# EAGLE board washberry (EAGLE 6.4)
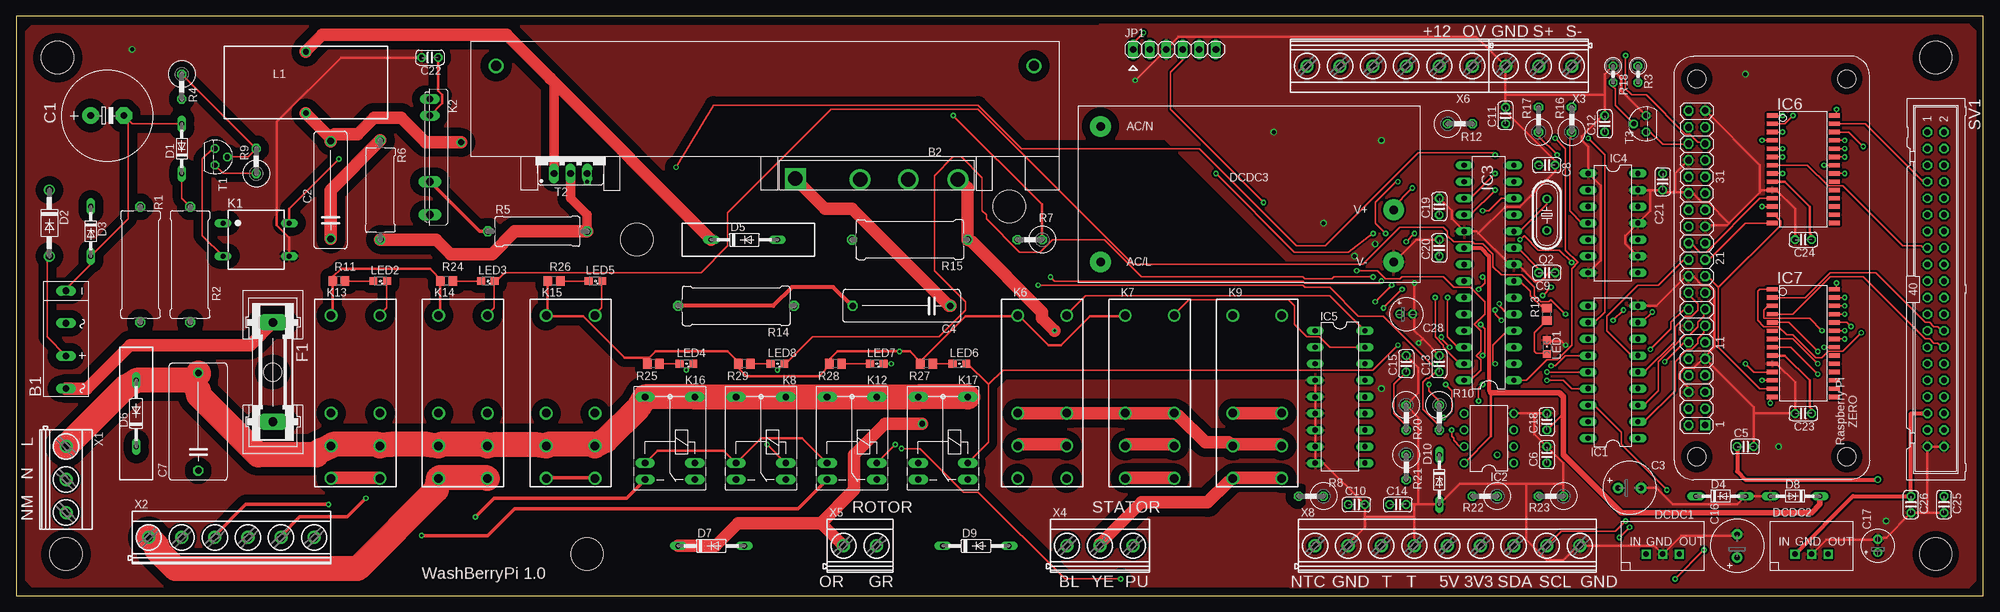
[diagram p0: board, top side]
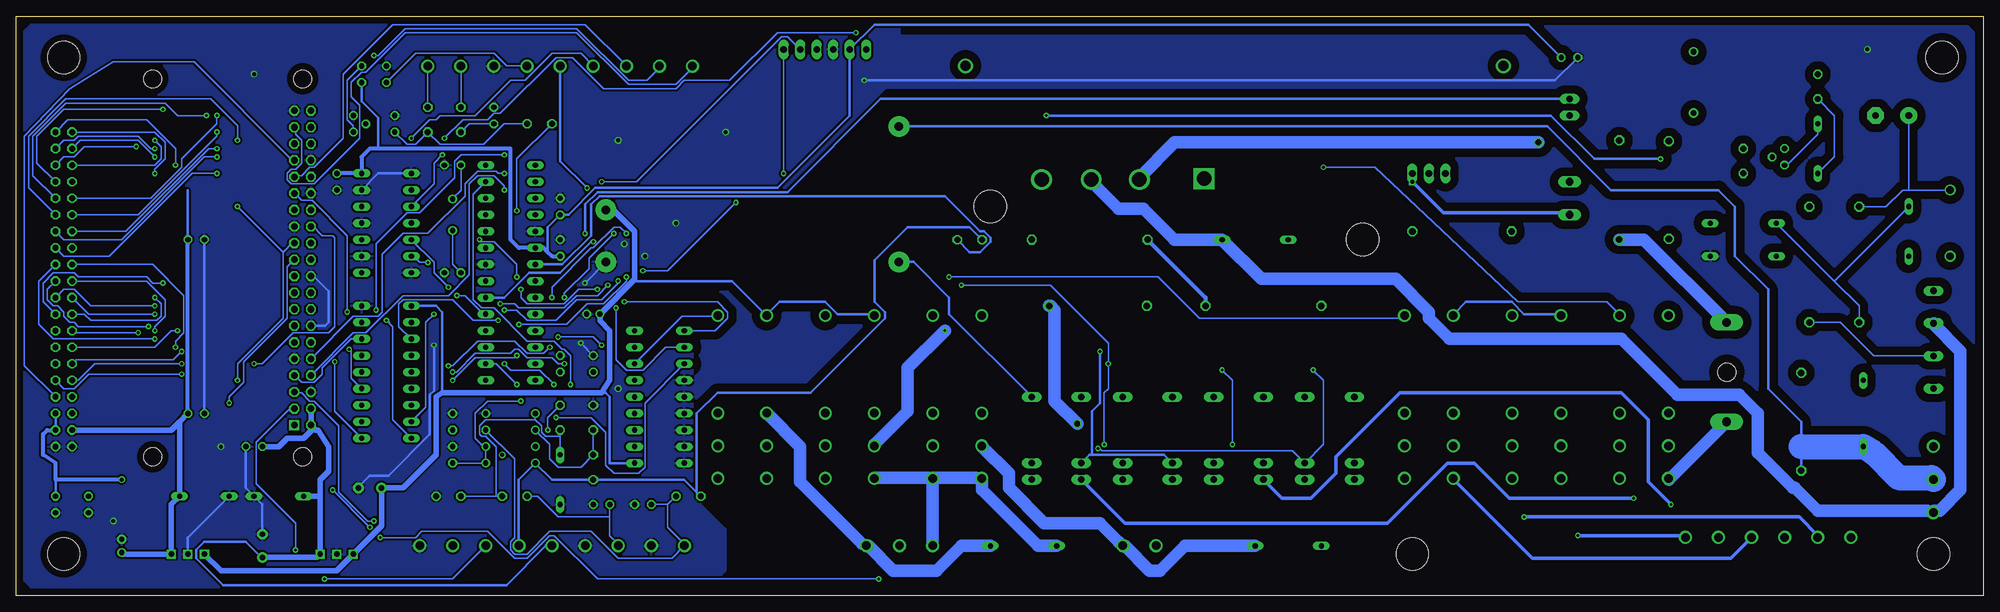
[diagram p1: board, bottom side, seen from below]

Size 301.93 x 88.89 mm. Coordinates in mm from the lower left corner, seen from the top.
Outline: 0,0 301.93,0 301.93,88.89 0,88.89 0,0
Copper layers (1*16): Top 0.035mm / dielectric 1.5mm / Bottom 0.035mm
Design rules "default *": minimum track width 5mil, minimum drill 0.4mm, track to track 6mil, track to pad 6mil, pad to pad 6mil, via to via 6mil, smd to smd 6mil, copper to edge 40mil, drill to drill 8mil, minimum pad ring 10mil, minimum via ring 8mil, stop-mask expansion 4mil, vias tented up to drill 0mil, thermal gap 10mil
Net classes: 0 default: width 0.254 mm; 1 10A: width 3.81 mm, drill 0.001 mm, clearance 1.016 mm; 2 5A: width 1.905 mm, drill 0.001 mm, clearance 1.016 mm; 3 2A: width 0.635 mm, drill 0.001 mm, clearance 1.016 mm; 4 0.5: width 0.508 mm, drill 0.001 mm, clearance 1.016 mm; 5 0.25: width 0.254 mm, clearance 1.016 mm; 6 12V: width 0.406 mm; 7 5V: width 0.406 mm; 8 3V3: width 0.406 mm; 9 small_signal: width 0.203 mm; 10 GND: width 0.406 mm; 11 TRIAC: width 0.406 mm
Holes 5 mm at 6.35,82.55 7.62,6.35 294.64,6.35 294.64,82.55 95.25,54.61 152.4,59.69 87.63,6.35

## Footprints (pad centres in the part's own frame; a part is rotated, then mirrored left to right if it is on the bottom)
2KBB = drill 1.016 long: + -2.616,0; - 7.391,0; AC1 -7.62,0; AC2 2.413,0
5S = drill 2.2 square: + 2.49,1.69 | drill 2.2: - 27.44,1.54; AC1 12.45,1.54; AC2 19.82,1.54
E5-13 = drill 1.016 pad 2.54: + -2.54,0 | drill 1.016 pad 2.54 octagon: - 2.54,0
C150-054X183 = drill 1.016 octagon: 1 -7.493,0; 2 7.493,0
E3,5-8 = drill 0.813 pad 1.6: + -1.778,0 | drill 0.813 pad 1.6 octagon: - 1.778,0
C025-024X044 = drill 0.813 octagon: 1 -1.27,0; 2 1.27,0
C150-091X182 = drill 1.016 octagon: 1 -7.493,0; 2 7.493,0
E2-5 = drill 0.813 pad 1.27: + -1.016,0 | drill 0.813 pad 1.27 octagon: - 1.016,0
DO34Z7 = drill 0.813 long: A 3.81,0; C -3.81,0
DO41-10 = drill 1.118: A 5.08,0; C -5.08,0
DO35-10 = drill 0.813 long: A 5.08,0; C -5.08,0
SIPTO220 = drill 0.813 pad 1.397 square: 1 -2.54,-1.27; 2 0,-1.27; 3 2.54,-1.27
IRM_15/20 = drill 1.3 pad 3.17: AC/L -22.8,-10.4; AC/N -22.8,10.4; V+ 22.2,-2.4; V- 22.2,-10.4
GSH15 = drill 1.321 pad 2.54 long: 1 -7.62,0; 2 7.62,0 | hole 2.794: 0,0
DIL18 = drill 0.813 long: 1 -10.16,-3.81; 2 -7.62,-3.81; 3 -5.08,-3.81; 4 -2.54,-3.81; 5 0,-3.81; 6 2.54,-3.81; 7 5.08,-3.81; 8 7.62,-3.81; 9 10.16,-3.81; 10 10.16,3.81; 11 7.62,3.81; 12 5.08,3.81; 13 2.54,3.81; 14 0,3.81; 15 -2.54,3.81; 16 -5.08,3.81; 17 -7.62,3.81; 18 -10.16,3.81
DIL08 = drill 0.813 pad 1.27: 1 -3.81,-3.81; 2 -1.27,-3.81; 3 1.27,-3.81; 4 3.81,-3.81; 5 3.81,3.81; 6 1.27,3.81; 7 -1.27,3.81; 8 -3.81,3.81
DIL28-3 = drill 0.813 long: 1 -16.51,-3.81; 2 -13.97,-3.81; 3 -11.43,-3.81; 4 -8.89,-3.81; 5 -6.35,-3.81; 6 -3.81,-3.81; 7 -1.27,-3.81; 8 1.27,-3.81; 9 3.81,-3.81; 10 6.35,-3.81; 11 8.89,-3.81; 12 11.43,-3.81; 13 13.97,-3.81; 14 16.51,-3.81; 15 16.51,3.81; 16 13.97,3.81; 17 11.43,3.81; 18 8.89,3.81; 19 6.35,3.81; 20 3.81,3.81; 21 1.27,3.81; 22 -1.27,3.81; 23 -3.81,3.81; 24 -6.35,3.81; 25 -8.89,3.81; 26 -11.43,3.81; 27 -13.97,3.81; 28 -16.51,3.81
DIL14 = drill 0.813 long: 1 -7.62,-3.81; 2 -5.08,-3.81; 3 -2.54,-3.81; 4 0,-3.81; 5 2.54,-3.81; 6 5.08,-3.81; 7 7.62,-3.81; 8 7.62,3.81; 9 5.08,3.81; 10 2.54,3.81; 11 0,3.81; 12 -2.54,3.81; 13 -5.08,3.81; 14 -7.62,3.81
SO28W = smd 0.65 x 1.7: 1 -7.62,-4.78; 2 -6.35,-4.78; 3 -5.08,-4.78; 4 -3.81,-4.78; 5 -2.54,-4.78; 6 -1.27,-4.78; 7 0,-4.78; 8 1.27,-4.78; 9 2.54,-4.78; 10 3.81,-4.78; 11 5.08,-4.78; 12 6.35,-4.78; 13 7.62,-4.78; 14 8.89,-4.78; 15 8.89,4.78; 16 7.62,4.78; 17 6.35,4.78; 18 5.08,4.78; 19 3.81,4.78; 20 2.54,4.78; 21 1.27,4.78; 22 0,4.78; 23 -1.27,4.78; 24 -2.54,4.78; 25 -3.81,4.78; 26 -5.08,4.78; 27 -6.35,4.78; 28 -7.62,4.78
1X06 = drill 1.016 long: 1 -6.35,0; 2 -3.81,0; 3 -1.27,0; 4 1.27,0; 5 3.81,0; 6 6.35,0
AQY27 = drill 0.8 long: 1 -2.54,-5.08; 2 2.54,-5.08; 3 2.54,5.08; 4 -2.54,5.08
AQZ-SIL04 = drill 1 long: 1 -8.89,0; 2 -6.35,0 | drill 1.2 long: 3 3.81,0; 4 8.89,0
FTR-K1C = drill 1.3 pad 1.93: 1 -12.5,-3.75; 2 2.5,-3.75; 3 7.5,-3.75; 4 12.5,-3.75; 5 12.5,3.75; 6 7.5,3.75; 7 2.5,3.75; 8 -12.5,3.75
M3XXH = drill 1.016 long: 1 -3.81,3.81; 2 -3.81,-3.81; O -6.35,-3.81; P 6.35,-3.81; P@ 6.35,3.81; S -6.35,3.81
TJ5-U1 = drill 0.9: 1 -4.7,0; 2 4.7,0
CHIPLED_0805 = smd 1.2 x 1.2: A 0,-1.05; C 0,1.05
SML0805 = smd 1.2 x 1.2: A 1.05,0; C -1.05,0
HC49/S = drill 0.813: 1 -2.413,0; 2 2.413,0
0617/17 = drill 1.016 octagon: 1 -8.89,0; 2 8.89,0
0207/2V = drill 0.813 octagon: 1 -1.27,0; 2 1.27,0
0411V = drill 0.914 octagon: 1 -2.54,0; 2 1.27,0
P0613/15 = drill 1.016 octagon: 1 -7.62,0; 2 7.62,0
R0805 = smd 1.3 x 1.5: 1 -0.95,0; 2 0.95,0
W_HEATSINK = drill 1.5: P$1 -40.64,5.08; P$2 41.91,5.08
ML40 = drill 0.914 octagon: 1 -24.13,-1.27; 2 -24.13,1.27; 3 -21.59,-1.27; 4 -21.59,1.27; 5 -19.05,-1.27; 6 -19.05,1.27; 7 -16.51,-1.27; 8 -16.51,1.27; 9 -13.97,-1.27; 10 -13.97,1.27; 11 -11.43,-1.27; 12 -11.43,1.27; 13 -8.89,-1.27; 14 -8.89,1.27; 15 -6.35,-1.27; 16 -6.35,1.27; 17 -3.81,-1.27; 18 -3.81,1.27; 19 -1.27,-1.27; 20 -1.27,1.27; 21 1.27,-1.27; 22 1.27,1.27; 23 3.81,-1.27; 24 3.81,1.27; 25 6.35,-1.27; 26 6.35,1.27; 27 8.89,-1.27; 28 8.89,1.27; 29 11.43,-1.27; 30 11.43,1.27; 31 13.97,-1.27; 32 13.97,1.27; 33 16.51,-1.27; 34 16.51,1.27; 35 19.05,-1.27; 36 19.05,1.27; 37 21.59,-1.27; 38 21.59,1.27; 39 24.13,-1.27; 40 24.13,1.27
TO92 = drill 0.813 octagon: 1 1.27,0; 2 0,1.905; 3 -1.27,0
TO220BV = drill 1.016 long: G 2.54,-2.54; T1 -2.54,-2.54; T2 0,-2.54
ZERO_NO_DIMENSION = drill 1.016 square: 1 8.37,25.24 | drill 1.016 octagon: 2 8.37,27.78; 3 10.91,25.24; 4 10.91,27.78; 5 13.45,25.24; 6 13.45,27.78; 7 15.99,25.24; 8 15.99,27.78; 9 18.53,25.24; 10 18.53,27.78; 11 21.07,25.24; 12 21.07,27.78; 13 23.61,25.24; 14 23.61,27.78; 15 26.15,25.24; 16 26.15,27.78; 17 28.69,25.24; 18 28.69,27.78; 19 31.23,25.24; 20 31.23,27.78; 21 33.77,25.24; 22 33.77,27.78; 23 36.31,25.24; 24 36.31,27.78; 25 38.85,25.24; 26 38.85,27.78; 27 41.39,25.24; 28 41.39,27.78; 29 43.93,25.24; 30 43.93,27.78; 31 46.47,25.24; 32 46.47,27.78; 33 49.01,25.24; 34 49.01,27.78; 35 51.55,25.24; 36 51.55,27.78; 37 54.09,25.24; 38 54.09,27.78; 39 56.63,25.24; 40 56.63,27.78 | hole 2.75: 3.5,3.5; 3.5,26.5; 61.5,26.5; 61.5,3.5
MKDSN1,5/3-5,08 = drill 1.3 pad 2: 1 -7.641,0.025; 2 -2.561,0.025; 3 2.519,0.025
MKDSN1,5/6-5,08 = drill 1.3 pad 2: 1 -12.7,0.025; 2 -7.62,0.025; 3 -2.54,0.025; 4 2.54,0.025; 5 7.62,0.025; 6 12.7,0.025
MKDSN1,5/2-5,08 = drill 1.3 pad 2: 1 -2.561,0.025; 2 2.519,0.025
MKDSN1,5/9-5,08 = drill 1.3 pad 2: 1 -20.341,0.025; 2 -15.261,0.025; 3 -10.181,0.025; 4 -5.101,0.025; 5 -0.021,0.025; 6 5.059,0.025; 7 10.139,0.025; 8 15.219,0.025; 9 20.299,0.025

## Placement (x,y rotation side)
B1  [2KBB]  7.62,39.37 90 top
B2  D15XB60  [5S]  117.1,62.3 0 top
C1  470µ  [E5-13]  13.97,73.66 0 top
C2  1nF  [C150-054X183]  48.26,62.23 90 top
C3  100µF  [E3,5-8]  247.65,16.51 0 top
C4  100nF  [C150-054X183]  135.89,44.45 180 top
C5  100nF  [C025-024X044]  265.43,22.86 0 top
C6  100nF  [C025-024X044]  234.95,21.59 90 top
C7  1nF  [C150-091X182]  27.94,26.67 90 top
C8  20pF  [C025-024X044]  234.95,66.04 0 top
C9  20pF  [C025-024X044]  234.95,49.53 0 top
C10  22nF  [C025-024X044]  205.74,13.97 0 top
C11  100nF  [C025-024X044]  228.6,73.66 90 top
C12  0  [C025-024X044]  243.84,72.39 90 top
C13  22pF  [C025-024X044]  218.44,35.56 90 top
C14  100nF  [C025-024X044]  212.09,13.97 0 top
C15  100nF  [C025-024X044]  213.36,35.56 90 top
C16  100µF  [E3,5-8]  264.16,7.62 90 top
C17  100µF  [E2-5]  285.75,7.62 90 top
C18  100nF  [C025-024X044]  234.95,26.67 90 top
C19  100nF  [C025-024X044]  218.44,59.69 90 top
C20  100nF  [C025-024X044]  218.44,53.34 90 top
C21  100nF  [C025-024X044]  252.73,63.5 270 top
C22  100nF  [C025-024X044]  63.5,82.55 180 top
C23  100nF  [C025-024X044]  274.32,27.94 180 top
C24  100nF  [C025-024X044]  274.32,54.61 180 top
C25  100nF  [C025-024X044]  295.91,13.97 270 top
C26  100nF  [C025-024X044]  290.83,13.97 270 top
C28  [E2-5]  213.36,43.18 0 top
D1  12V  [DO34Z7]  25.4,68.58 90 top
D2  1N4004  [DO41-10]  5.08,57.15 270 top
D3  5V  [DO34Z7]  11.43,55.88 270 top
D4  5V8  [DO34Z7]  261.62,15.24 0 top
D5  [DO35-10]  111.76,54.61 0 top
D6  [DO35-10]  18.41,27.94 90 top
D7  [DO35-10]  106.68,7.62 0 top
D8  3V6  [DO34Z7]  273.05,15.24 180 top
D9  [DO35-10]  147.32,7.62 0 top
D10  3V3  [DO34Z7]  218.44,17.78 270 top
DCDC1  TSR1-2405  [SIPTO220]  252.73,7.62 0 top
DCDC2  TSR1-2405  [SIPTO220]  275.59,7.62 0 top
DCDC3  IRM-15-12  [IRM_15/20]  189.23,61.59 0 top
F1  5A  [GSH15]  39.37,34.29 270 top
IC1  ULN2803  [DIL18]  245.11,34.29 90 top
IC2  LM358N  [DIL08]  226.06,24.13 90 top
IC3  PIC18F2550_28DIP  [DIL28-3]  226.06,49.53 90 top
IC4  74HC04N  [DIL14]  245.11,57.15 270 top
IC5  ULN2803  [DIL18]  203.2,30.48 270 top
IC6  MCP23S17SO  [SO28W]  274.32,66.04 270 top
IC7  MCP23S17SO  [SO28W]  274.32,39.37 270 top
JP1  ISCP  [1X06]  177.8,83.82 0 top
K1  AQYAQY27  [AQY27]  36.83,54.61 270 top
K2  AQZ204  [AQZ-SIL04]  63.5,67.31 270 top
K6  FTR-K1C  [FTR-K1C]  157.48,30.48 270 top
K7  FTR-K1C  [FTR-K1C]  173.99,30.48 270 top
K8  M3XXH  [M3XXH]  114.3,24.13 90 top
K9  FTR-K1C  [FTR-K1C]  190.5,30.48 270 top
K12  M3XXH  [M3XXH]  128.27,24.13 90 top
K13  FTR-K1C  [FTR-K1C]  52.07,30.48 270 top
K14  FTR-K1C  [FTR-K1C]  68.58,30.48 270 top
K15  FTR-K1C  [FTR-K1C]  85.09,30.48 270 top
K16  M3XXH  [M3XXH]  100.33,24.13 90 top
K17  M3XXH  [M3XXH]  142.24,24.13 90 top
L1  [TJ5-U1]  44.45,78.74 270 top
LED1  [CHIPLED_0805]  234.95,38.1 0 top
LED2  [SML0805]  55.88,48.26 180 top
LED3  [SML0805]  72.39,48.26 180 top
LED4  [SML0805]  102.87,35.56 180 top
LED5  [SML0805]  88.9,48.26 180 top
LED6  [SML0805]  144.78,35.56 180 top
LED7  [SML0805]  132.08,35.56 180 top
LED8  [SML0805]  116.84,35.56 180 top
Q2  12MHz  [HC49/S]  234.95,58.42 270 top
R1  82K  [0617/17]  19.05,50.8 270 top
R2  47K  [0617/17]  26.67,50.8 270 top
R3  10K  [0207/2V]  248.92,80.01 270 top
R4  1K  [0411V]  25.4,77.47 270 top
R5  470  [P0613/15]  80.01,55.88 0 top
R6  68  [P0613/15]  55.88,62.23 270 top
R7  1K  [0411V]  154.94,54.61 180 top
R8  10K  [0411V]  198.12,15.24 180 top
R9  47K  [0411V]  36.83,67.31 90 top
R10  10K  [0411V]  218.44,26.67 270 top
R11  [R0805]  49.53,48.26 180 top
R12  1K  [0411V]  222.25,72.39 0 top
R13  1K  [R0805]  234.95,43.18 90 top
R14  68  [0617/17]  110.49,44.45 180 top
R15  68  [0617/17]  137.16,54.61 180 top
R16  0  [0411V]  238.76,73.66 90 top
R17  0  [0411V]  233.68,73.66 90 top
R18  470K  [0207/2V]  245.11,80.01 270 top
R20  1K  [0411V]  213.36,26.67 270 top
R21  8K2  [0411V]  213.36,19.05 270 top
R22  1K  [0411V]  224.79,15.24 180 top
R23  47K  [0411V]  234.95,15.24 180 top
R24  [R0805]  66.04,48.26 180 top
R25  [R0805]  97.79,35.56 180 top
R26  [R0805]  82.55,48.26 180 top
R27  [R0805]  139.7,35.56 180 top
R28  [R0805]  125.73,35.56 180 top
R29  [R0805]  111.76,35.56 180 top
SINK1  HEATSINK  [W_HEATSINK]  114.3,76.2 0 top
SV1  [ML40]  294.64,46.99 270 top
T1  BC547  [TO92]  30.48,67.31 270 top
T2  BTA25-6CWG  [TO220BV]  85.09,67.31 0 top
T3  BC547  [TO92]  250.19,72.39 90 top
U$3  ZERO  [ZERO_NO_DIMENSION]  284.48,17.78 90 top
X1  [MKDSN1,5/3-5,08]  7.62,15.24 270 top
X2  MKDSN1,5/6-5,08  [MKDSN1,5/6-5,08]  33.02,8.89 0 top
X3  MKDSN1,5/3-5,08  [MKDSN1,5/3-5,08]  231.14,81.28 180 top
X4  MKDSN1,5/3-5,08  [MKDSN1,5/3-5,08]  168.91,7.62 0 top
X5  MKDSN1,5/2-5,08  [MKDSN1,5/2-5,08]  129.54,7.62 0 top
X6  MKDSN1,5/6-5,08  [MKDSN1,5/6-5,08]  210.82,81.28 180 top
X8  MKDSN1,5/9-5,08  [MKDSN1,5/9-5,08]  219.71,7.62 0 top

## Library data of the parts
B1 = rectifier
B2 = D15XB60
C1-C26 C28 L1 R1-R18 R20-R29 = rcl
D1-D10 = diode
DCDC1 DCDC2 = TSR1-24XX
DCDC3 = meanwell_irm_v7
F1 = fuse; MPN: 64900001039; OC_FARNELL: 1271673; OC_NEWARK: 02P0318
IC1 IC5 = uln-udn
IC2 = linear
IC3 = microchip; MF: MICROCHIP; MPN: PIC18F2550-I/SP; OC_FARNELL: 1523822; OC_NEWARK: 80K6054
IC4 = 74xx-eu
IC6 IC7 = microchip; MF: MICROCHIP; MPN: MCP23S17-E/SO; OC_FARNELL: unknown; OC_NEWARK: 31K2950
JP1 = pinhead
K1 K6-K9 K12-K17 = relay; OC_FARNELL: unknown; OC_NEWARK: unknown
K2 = relay; MPN: AQZ204; OC_FARNELL: unknown; OC_NEWARK: 13P1222
LED1-LED8 = led
Q2 = crystal; OC_FARNELL: 1667008; OC_NEWARK: unknown
SINK1 = Heatsink_Washmachine
SV1 = con-harting-ml; OC_FARNELL: unknown; OC_NEWARK: unknown
T1 T3 = transistor
T2 = triac
U$3 = RasPiZero
X1 X3 X4 = con-phoenix-508; MPN: SMKDSN1,5/3-5,08; OC_FARNELL: 1792904; OC_NEWARK: 70R0299
X2 X6 = con-phoenix-508; MPN: SMKDSN1,5/6-5,08; OC_FARNELL: 1792907; OC_NEWARK: 70R0302
X5 = con-phoenix-508; MPN: MKDSN 1,5/2-5.08; OC_FARNELL: 1792903; OC_NEWARK: 30M2397
X8 = con-phoenix-508; MPN: SMKDSN1,5/9-5,08; OC_FARNELL: 1792912; OC_NEWARK: 70R0305

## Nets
+3V3 [3V3]: C17.+ C18.1 C19.1 C20.1 C21.1 C22.1 C23.1 C24.1 D8.C DCDC2.3 IC2.8 IC3.20 IC4.14 IC6.9 IC7.9 JP1.2 K2.2 R3.2 R7.2 R8.2 R21.2 SV1.37 X8.6
+5V [5V]: C5.1 C16.+ C25.1 D4.C DCDC1.3 SV1.36 SV1.38 U$3.2 U$3.4 X8.5
+12V [12V]: C3.+ C26.1 C28.+ DCDC1.1 DCDC2.1 DCDC3.V+ IC1.10 IC5.10 K6.1 K7.1 K8.1 K9.1 K12.1 K13.1 K14.1 K15.1 K16.1 K17.1 R11.2 R24.2 R25.2 R26.2 R27.2 R28.2 R29.2 SV1.35 X6.2
BOOST [small_signal]: IC3.4 IC5.3
CS0: IC6.11 U$3.24
CS1: IC7.11 U$3.26
DIRECTION [small_signal]: IC3.5 IC4.5 IC5.1
GND [GND]: C3.- C5.2 C6.2 C8.2 C9.2 C10.2 C11.2 C12.2 C13.2 C14.2 C15.2 C16.- C17.- C18.2 C19.2 C20.2 C21.2 C22.2 C23.2 C24.2 C25.2 C26.2 C28.- D4.A D8.A D10.A DCDC1.2 DCDC2.2 DCDC3.V- IC1.9 IC2.4 IC3.8 IC3.19 IC4.1 IC4.7 IC4.9 IC4.11 IC4.13 IC5.4 IC5.5 IC5.6 IC5.7 IC5.8 IC5.9 IC6.10 IC7.10 JP1.3 K1.3 LED1.C R18.1 R20.1 R23.1 SV1.39 SV1.40 T3.1 U$3.6 U$3.9 U$3.14 U$3.20 U$3.25 U$3.30 U$3.34 U$3.39 X3.3 X8.2 X8.4 X8.9
GPA1.0: IC6.21 SV1.1
GPA1.1: IC6.22 SV1.2
GPA1.2: IC6.23 SV1.3
GPA1.3: IC6.24 SV1.4
GPA1.4: IC6.25 SV1.5
GPA1.5: IC6.26 SV1.6
GPA1.6: IC6.27 SV1.7
GPA1.7: IC6.28 SV1.8
GPA2.0: IC7.21 SV1.17
GPA2.1: IC7.22 SV1.18
GPA2.2: IC7.23 SV1.19
GPA2.3: IC7.24 SV1.20
GPA2.4: IC7.25 SV1.21
GPA2.5: IC7.26 SV1.22
GPA2.6: IC7.27 SV1.23
GPA2.7: IC7.28 SV1.24
GPB1.0: IC6.1 SV1.9
GPB1.1: IC6.2 SV1.10
GPB1.2: IC6.3 SV1.11
GPB1.3: IC6.4 SV1.12
GPB1.4: IC6.5 SV1.13
GPB1.5: IC6.6 SV1.14
GPB1.6: IC6.7 SV1.15
GPB1.7: IC6.8 SV1.16
GPB2.0: IC7.1 SV1.25
GPB2.1: IC7.2 SV1.26
GPB2.2: IC7.3 SV1.27
GPB2.3: IC7.4 SV1.28
GPB2.4: IC7.5 SV1.29
GPB2.5: SV1.30
GPB2.6: IC7.7 SV1.31
GPB2.7: IC7.8 SV1.32
GPIO0: U$3.11
GPIO1 [small_signal]: IC1.1 U$3.12
GPIO2 [small_signal]: IC1.2 U$3.13
GPIO3 [small_signal]: IC1.3 U$3.15
GPIO4 [small_signal]: IC1.4 U$3.16
GPIO5 [small_signal]: IC1.5 U$3.18
GPIO6 [small_signal]: IC1.6 U$3.22
GPIO7 [small_signal]: IC1.7 U$3.7
GPIO21 [small_signal]: IC1.8 U$3.29
GPIO27 [small_signal]: R3.1 T3.3 U$3.36
GPPB2.5: IC7.6
INT [TRIAC]: IC3.21 K1.4 R7.1
L [10A]: C7.2 D6.A DCDC3.AC/L K8.P K8.P@ K12.P K12.P@ K13.3 K13.6 K14.3 K14.6 K15.3 K15.6 K16.P K16.P@ K17.P K17.P@ X1.1
L-MOTOR [5A]: F1.2 K13.4 K13.5
MISO: IC6.14 IC7.14 U$3.21
MOSI: IC6.13 IC7.13 U$3.19
N [10A]: C7.1 D6.C DCDC3.AC/N X1.2
N$1 [0.25]: K1.2 T1.3
N$2 [0.25]: B1.- C1.- D1.A D3.A R9.1 T1.1
N$3 [0.25]: C1.+ D2.C R1.1
N$4 [0.25]: D3.C K1.1 R1.2
N$5 [small_signal]: IC3.7 R13.2
N$6 [small_signal]: LED1.A R13.1
N$7 [0.25]: D1.C R2.1 R4.2
N$8: IC1.11 X6.3
N$9 [0.25]: R4.1 R9.2 T1.2
N$10 [0.25]: B1.+ D2.A R2.2
N$11 [small_signal]: R18.2 T3.2 X6.1
N$12 [0.5]: K2.4 T2.G
N$13 [0.5]: K2.3 R5.1
N$14: IC2.7 IC3.13 R10.1
N$15: IC1.18 K13.8 LED2.C
N$16 [5A]: B2.- K7.3 K7.6 R15.1
N$17 [5A]: C2.1 R6.1
N$18 [5A]: B2.AC1 C2.2 L1.2
N$19: C6.1 IC2.1 IC2.2 IC3.2
N$20 [5A]: K9.4 K9.5 X4.2
N$21 [5A]: D9.A K9.2 K9.7 X4.3
N$22: LED2.A R11.1
N$23 [5A]: D5.C L1.1 T2.T1
N$24 [5A]: B2.+ C4.1 D7.C X5.1
N$25 [small_signal]: C9.1 IC3.9 Q2.2
N$26 [small_signal]: C8.1 IC3.10 Q2.1
N$27 [small_signal]: IC3.12 R12.1
N$28: C11.1 IC4.3 R17.1
N$29: C12.1 IC4.4 R12.2 R16.1
N$30: IC1.17 K14.8 LED3.C
N$31 [2A]: R14.1 R15.2
N$32 [2A]: C4.2 R14.2
N$33 [5A]: K6.2 K6.7 K7.2 K7.7 K9.3 K9.6
N$34 [5A]: D9.C K6.4 K6.5 K7.4 K7.5 X4.1
N$35 [5A]: D7.A K6.3 K6.6 X5.2
N$36: IC5.18 K6.8
N$37: R16.2 X3.1
N$38: R17.2 X3.2
N$39: C15.1 IC2.6 R20.2 R21.1
N$40: LED3.A R24.1
N$41: C13.1 D10.C IC2.5 R10.2 R22.1 R23.2
N$42: IC1.16 K16.2 LED4.C
N$43: U$3.31 X6.4
N$44: U$3.35 X6.5
N$45: LED4.A R25.1
N$46: LED5.A R26.1
N$49: IC1.13 K17.2 LED6.C
N$50: LED6.A R27.1
N$51: IC1.14 K12.2 LED7.C
N$52: LED7.A R28.1
N$53: IC1.15 K8.2 LED8.C
N$54: LED8.A R29.1
N$55: IC1.12 K15.8 LED5.C
N$56: SV1.33
N$57 [small_signal]: IC4.6 IC5.2
N$58: U$3.37 X6.6
N$60: IC5.17 K7.8
N$62: IC5.16 K9.8
N$63 [10A]: K14.4 K14.5 X2.1
N$64 [0.5]: K16.S X2.2
N$65 [0.5]: K8.S X2.3
N$66 [0.5]: K12.S X2.6
N$67 [0.5]: K17.S X2.5
N$68 [0.5]: K15.4 K15.5 X2.4
N_MOTOR [5A]: B1.AC2 B2.AC2 D5.A X1.3
NTC: C10.1 IC2.3 R8.1 X8.1
PGC [small_signal]: IC3.27 JP1.5
PGD [small_signal]: IC3.28 JP1.4
PGM [small_signal]: IC3.26 JP1.6
PWM0: U$3.32
PWM1: SV1.34 U$3.33
RX: IC3.18 U$3.8
SCK: IC6.12 IC7.12 U$3.23
SCL: U$3.5 X8.8
SDA: U$3.3 X8.7
SUPPLY_MOTOR [5A]: B1.AC1 F1.1 R5.2 R6.2 T2.T2
TACHO: C14.1 R22.2 X8.3
TRIAC [TRIAC]: IC3.6 K2.1
TX: IC3.17 U$3.10
VPP [small_signal]: IC3.1 JP1.1

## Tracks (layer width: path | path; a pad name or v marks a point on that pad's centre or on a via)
+3V3
  Top 0.406: 226.38,31.11 226.38,24.45 IC2.8 | C22.1 64.77,77.47 65.41,76.83 65.41,75.56 K2.2 | IC7.9 271.46,36.83 275.27,33.02 275.27,28.89 275.59,28.57 C23.1 | IC6.9 271.46,63.5 275.27,59.69 275.27,55.56 275.59,55.24 C24.1 | C18.1 237.17,27.62 237.49,27.62
  Top 0.61: IC3.20 224.79,53.34 226.06,52.07 226.06,31.43 226.38,31.11
  Top 0.813: 226.38,31.11 236.85,31.11 237.49,30.48 237.49,27.62 237.49,21.59 246.38,12.7 275.59,12.7 276.86,13.97 D8.C
  Bottom 0.406: C24.1 275.59,62.23 | 197.49,15.88 199.39,17.78 R21.2 219.71,17.78 IC2.8 224.79,17.78 224.79,7.94 X8.6 | 197.49,15.88 R8.2 | R7.2 155.57,56.52 165.1,56.52 170.18,51.44 170.18,45.09 168.59,43.5 168.59,42.55 180.02,31.11 194.31,31.11 197.49,27.94 197.49,15.88 | 220.5,52.86 220.34,53.02 220.34,56.52 C19.1 217.17,58.42 213.04,62.55 185.1,62.55 173.99,73.66 JP1.2 170.18,87.63 69.85,87.63 C22.1 | R3.2 248.92,75.88 246.38,73.34 246.38,68.58
  Bottom 0.61: C23.1 C24.1 | C20.1 219.71,52.07 220.5,52.86 220.98,53.34 IC3.20 224.79,53.34 226.06,54.61 226.06,68.58 246.38,68.58 247.65,68.58 248.92,67.31 IC4.14 C21.1
  Bottom 0.813: C17.+ 285.5,6.35 DCDC2.3 278.13,13.97 D8.C 276.86,26.67 | SV1.37 278.13,25.4 276.86,26.67 | 276.86,26.67 C23.1
+5V  (via drill 0.6)
  Top 0.61: C5.1 264.16,19.05 265.43,17.78 v285.75,17.78
  Bottom 0.406: 295.91,17.78 C25.1 | SV1.38 SV1.36 | X8.5 219.71,7.62 220.66,7.62 226.69,1.59 270.19,1.59 274.32,5.71 274.32,6.99 273.05,8.26 266.7,8.26 264.48,6.03 C16.+
  Bottom 0.61: v285.75,17.78 295.91,17.78 295.91,20.32 297.81,21.59 297.81,24.77 297.18,25.4 SV1.38
  Bottom 0.813: 255.27,15.24 DCDC1.3 255.78,5.84 C16.+ | D4.C 255.27,15.24 | 255.27,15.24 255.27,17.78 254,19.05 254,22.86 255.59,25.4 255.95,25.4 256.25,25.7 | 256.25,25.7 U$3.2 U$3.4 | C5.1 261.62,22.86 260.35,24.13 257.81,24.13 256.25,25.7
+12V  (via drill 0.4)
  Top 0.406: R11.2 48.58,43.18 K13.1 | K14.1 65.09,43.18 R24.2 65.41,48.26 63.5,50.16 49.85,50.16 48.58,48.9 R11.2 | R11.2 | R26.2 81.6,43.18 K15.1 81.6,42.86 87,42.86 93.34,36.51 97.16,36.51 | 97.16,36.51 98.11,37.47 109.22,37.47 111.12,35.56 R29.2 110.81,34.92 112.08,33.66 123.19,33.66 125.09,35.56 R28.2 124.78,36.2 126.05,37.47 v135.57,37.47 137.16,37.47 138.75,35.88 | 97.16,36.51 96.84,36.2 R25.2 | K16.1 98.42,22.23 108.58,22.23 K8.1 114.3,24.13 120.65,24.13 K12.1 | v214.31,62.55 211.14,59.37 DCDC3.V+ | 138.75,35.88 139.06,35.56 R27.2 138.75,35.88 | 138.75,35.88 145.73,42.86 153.67,42.86 K6.1 153.99,42.86 158.43,38.42 160.34,38.42 164.78,42.86 170.18,42.86 K7.1
  Top 0.61: DCDC2.1 281.94,15.24 C26.1 290.83,27.94 SV1.35
  Bottom 0.406: 236.54,31.11 236.54,43.5 237.49,44.45 IC1.10 | 212.09,31.11 211.46,31.11 210.82,30.48 210.82,20.32 IC5.10 | K14.1 65.09,43.18 70.48,43.18 72.39,45.09 79.38,45.09 81.28,43.18 K15.1 | K17.1 137.16,21.59 136.84,21.59 | 136.84,21.59 125.73,21.59 K12.1 | X6.2 218.44,66.67 v214.31,62.55 | K7.1 170.5,43.18 175.9,43.18 177.8,45.09 184.78,45.09 186.69,43.18 K9.1 187.01,43.18 192.09,48.26 206.69,48.26 207.01,48.51 | 136.84,21.59 136.84,28.26 135.57,29.53 v135.57,37.47
  Bottom 0.813: DCDC3.V+ 210.32,59.2 207.01,55.88 207.01,48.51 C28.+ 212.34,42.16 210.82,40.64 210.82,33.02 212.09,31.11 236.54,31.11 237.49,30.48 237.49,21.59 242.57,16.51 C3.+ 245.87,10.67 DCDC1.1 252.73,3.81 270.51,3.81 DCDC2.1
BOOST  (via drill 0.4)
  Top 0.203: v219.07,27.3 219.39,27.3 220.34,28.26 220.34,31.43 v219.39,32.38 | v227.01,35.56 226.69,35.88 226.69,38.42 228.92,40.64 IC3.4
  Bottom 0.203: IC5.3 205.42,29.53 205.42,19.68 206.38,18.73 210.19,18.73 211.46,20 211.46,25.08 213.68,27.3 v219.07,27.3 | v219.39,32.38 221.62,34.61 226.06,34.61 v227.01,35.56
CS0
  Top 0.254: IC6.11 267.65,60.96 259.4,52.7 258.44,52.7 256.86,54.29 U$3.24
CS1  (via drill 0.4)
  Top 0.254: IC7.11 266.7,34.29 v265.43,35.56
  Bottom 0.254: v265.43,35.56 264.16,35.56 259.4,40.32 254,40.32 253.05,41.27 253.05,54.93 253.37,55.24 254.95,55.24 256.54,56.83 U$3.26
DIRECTION  (via drill 0.4)
  Top 0.203: v211.14,47.62 v208.6,45.09 | v227.65,44.77 227.65,44.45 228.92,43.18 IC3.5 | v234.31,46.04 v235.59,47.31
  Bottom 0.203: IC5.1 194.63,40.64 192.72,42.55 192.72,43.5 194.31,45.09 v208.6,45.09 | v211.14,47.62 212.72,46.04 215.9,46.04 217.81,44.13 224.79,44.13 225.43,44.77 v227.65,44.77 | IC4.5 237.81,51.12 237.81,49.53 v235.59,47.31 | v234.31,46.04 233.04,46.04 230.19,43.18 IC3.5
GND  (via drill 0.4, 0.6)
  Top 0.406: C18.2 233.04,27.94 | 233.04,27.94 IC2.4 | 233.04,27.94 233.04,24.77 C6.2 237.49,20.32 237.49,17.14 | 237.49,17.14 R23.1 | C20.2 214.95,54.61 211.46,51.12 DCDC3.V- | IC5.4 IC5.5 IC5.6 IC5.7 IC5.8 IC5.9 200.66,20.32 C10.2 207.01,12.06 | 207.01,12.06 207.01,10.48 204.47,7.94 X8.2 | 214.63,43.18 214.63,40.64 215.9,39.37 | C13.2 215.9,39.37 | C15.2 215.26,34.92 215.26,31.11 R20.1 215.26,27.3 215.26,13.97 | 215.26,13.97 D10.A 221.62,17.14 231.78,17.14 | 215.26,13.97 214.63,13.97 | 214.63,13.97 C14.2 | 214.63,13.97 214.63,12.06 | 214.63,12.06 214.63,7.94 X8.4 | v215.26,38.73 215.9,39.37 | 214.63,12.06 207.01,12.06 | 214.63,43.18 v214.63,47.94 | 214.63,43.18 C28.- | 231.78,17.14 237.49,17.14 | v237.81,38.42 237.17,39.05 234.95,39.05 LED1.C | C16.- 264.16,9.21 255.59,9.21 DCDC1.2 251.46,7.62 240.03,7.62 X8.9 239.71,7.62 237.49,5.4 234.95,5.4 231.78,8.57 231.78,17.14 | SV1.40 SV1.39 293.37,12.7 | 293.37,12.7 C26.2 287.02,8.89 285.75,8.89 C17.- 285.75,8.57 277.81,8.57 DCDC2.2 | 293.37,12.7 C25.2 | IC1.9 251.78,44.45 256.54,49.21 U$3.20 256.86,48.9 257.49,48.9 258.76,47.62 259.71,47.62 260.67,46.67 260.67,38.1 259.08,36.51 | IC7.10 270.19,35.56 273.05,32.7 C23.2 266.7,27.94 | 259.08,36.51 257.49,34.92 256.22,34.92 255.27,33.97 255.27,33.34 256.54,32.07 256.54,31.43 U$3.6 | D8.A D4.A 264.16,13.97 254.32,13.97 251.78,16.51 C3.- | C5.2 266.7,27.94 | 266.7,27.94 266.7,28.89 259.4,36.2 U$3.9 259.08,36.51 | IC4.7 243.21,51.44 243.21,62.87 IC4.1 241.3,68.9 240.35,69.85 240.35,70.48 243.84,73.98 | IC4.9 247.01,53.98 247.01,55.24 IC4.11 250.82,59.05 250.82,62.23 | 250.82,62.23 C21.2 253.05,61.91 254.63,61.91
  Top 0.406: 250.82,62.23 IC4.13 | 254.63,61.91 256.54,61.91 U$3.30 256.86,61.59 257.49,61.59 258.76,60.33 259.71,60.33 262.89,57.15 | 254.63,61.91 254.63,64.77 256.54,66.67 U$3.34 | C24.2 273.05,59.37 270.19,62.23 IC6.10 267.97,62.23 267.65,61.91 | 267.65,61.91 262.89,57.15 | 262.89,57.15 262.57,56.83 259.4,56.83 U$3.25 | 267.65,61.91 267.65,66.04 259.4,74.3 U$3.39 | K1.3 41.91,54.93 40.01,56.83 40.01,72.71 49.85,82.55 C22.2 | C19.2 220.34,59.05 220.34,57.78 IC3.19 224.16,55.88 224.47,55.56 | 224.47,55.56 229.24,50.8 IC3.8 230.5,50.8 233.04,48.26 234,48.26 235.27,49.53 C9.2 | 243.84,76.83 243.84,80.01 244.79,80.96 | 243.84,76.83 243.84,73.98 | T3.1 246.38,77.47 246.38,79.38 244.79,80.96 | 244.79,80.96 R18.1 | 228.6,76.83 228.6,80.96 X3.3 228.6,81.28 224.16,85.72 178.44,85.72 JP1.3 v171.77,79.06 | 228.6,76.83 C11.2 228.6,74.3 236.22,66.67 C8.2 236.22,65.09 230.82,59.69 228.6,59.69 224.47,55.56 | 228.6,76.83 243.84,76.83 | 243.84,73.98 C12.2
  Bottom 0.406: C15.2 v215.26,38.73 | v214.63,47.94 211.46,51.12 DCDC3.V- | v237.81,38.42 237.81,31.43 238.44,30.8 238.44,24.77 244.79,18.41 247.65,18.41 249.56,16.51 C3.- | C5.2 266.7,16.51 D4.A 264.16,13.97 C16.- | DCDC2.2 275.59,8.89 D8.A | IC4.1 246.38,64.77 IC4.13 | C22.2 65.72,79.06 v171.77,79.06 | C24.2 C23.2 | U$3.14 254.52,41.39 254,41.91 254,46.67 256.22,48.9 256.58,48.9 U$3.20
  other vias: 193.04,71.12 209.55,69.85 265.43,80.01 270.51,22.86 287.02,11.43 209.55,31.75 17.78,83.82 200.66,57.15 205.42,52.07 208.6,53.98
  pour Bottom (isolate 1.27): 1.27,86.36 2.54,87.63 299.72,87.63 300.99,86.36 300.99,2.54 299.72,1.27 2.54,1.27 1.27,2.54
  pour Top (isolate 1.27): 1.27,86.36 2.54,87.63 299.72,87.63 300.99,86.36 300.99,2.54 299.72,1.27 2.54,1.27 1.27,2.54
  pour Bottom (isolate 0.305): 166.37,82.55 166.37,87.63 299.72,87.63 300.99,86.36 300.99,2.54 299.72,1.27 195.58,1.27 193.04,3.81 193.04,10.16 198.12,15.24 198.12,48.26 166.37,80.01
  pour Top (isolate 0.305): 166.37,80.01 166.37,87.63 299.72,87.63 300.99,86.36 300.99,2.54 299.72,1.27 195.58,1.27 194.31,2.54 194.31,10.16 198.12,13.97 198.12,48.26 196.85,49.53
GPA1.0  (via drill 0.4)
  Top 0.254: v280.67,64.77 IC6.21
  Bottom 0.254: v280.67,64.77 280.67,65.41 279.08,66.99 279.08,69.53 280.67,71.12 SV1.1
GPA1.1  (via drill 0.4)
  Top 0.254: v277.5,66.04 IC6.22
  Bottom 0.254: v277.5,66.04 277.5,68.58 281.94,73.03 294,73.03 SV1.2
GPA1.2  (via drill 0.4)
  Top 0.254: v280.67,67.31 IC6.23
  Bottom 0.254: v280.67,67.31 283.21,69.85 292.1,69.85 SV1.3
GPA1.3  (via drill 0.4)
  Top 0.254: v280.67,68.58 IC6.24
  Bottom 0.254: v280.67,68.58 281.31,68.58 283.21,70.48 292.42,70.48 293.05,69.85 294.64,69.85 SV1.4
GPA1.4  (via drill 0.4)
  Top 0.254: v280.67,69.85 IC6.25
  Bottom 0.254: v280.67,69.85 279.72,68.9 279.72,66.99 280.67,66.04 SV1.5
GPA1.5  (via drill 0.4)
  Top 0.254: IC6.26 281.31,71.12 v283.53,68.9
  Bottom 0.254: v283.53,68.9 291.46,68.9 293.05,67.31 294.64,67.31 SV1.6
GPA1.6
  Top 0.254: IC6.27 283.85,72.39 292.74,63.5 SV1.7
GPA1.7  (via drill 0.4)
  Top 0.254: v279.4,74.61 279.4,73.66 IC6.28
  Bottom 0.254: v279.4,74.61 294.64,74.61 298.77,70.48 298.77,66.36 SV1.8
GPA2.0  (via drill 0.4)
  Top 0.254: v277.5,38.1 IC7.21
  Bottom 0.254: v277.5,38.1 277.5,39.05 276.23,40.32 276.23,46.04 280.99,50.8 SV1.17
GPA2.1  (via drill 0.4)
  Top 0.254: v280.67,39.37 IC7.22
  Bottom 0.254: v280.67,39.37 296.23,39.37 298.45,41.59 298.45,48.26 SV1.18
GPA2.2  (via drill 0.4)
  Top 0.254: v280.67,40.64 IC7.23
  Bottom 0.254: v280.67,40.64 280.67,41.27 279.08,42.86 279.08,45.4 281.94,48.26 SV1.19
GPA2.3  (via drill 0.4)
  Top 0.254: IC7.24 280.99,41.91 v281.62,41.27
  Bottom 0.254: v281.62,41.27 292.42,41.27 293.05,41.91 293.69,41.91 294.64,42.86 294.64,43.5 295.59,44.45 296.23,44.45 297.18,45.4 297.18,46.99 SV1.20
GPA2.4  (via drill 0.4)
  Top 0.254: v280.67,43.18 IC7.25
  Bottom 0.254: v280.67,43.18 290.83,43.18 SV1.21
GPA2.5  (via drill 0.4)
  Top 0.254: v280.67,44.45 IC7.26
  Bottom 0.254: v280.67,44.45 290.51,44.45 293.05,46.99 294.64,46.99 SV1.22
GPA2.6  (via drill 0.4)
  Top 0.254: v280.67,45.72 IC7.27
  Bottom 0.254: v280.67,45.72 279.72,44.77 279.72,42.86 280.35,42.23 290.51,42.23 291.46,43.18 SV1.23
GPA2.7  (via drill 0.4)
  Top 0.254: v279.4,47.94 279.4,46.99 IC7.28
  Bottom 0.254: v279.4,47.94 280.99,47.94 281.94,48.9 292.42,48.9 293.05,49.53 296.23,49.53 297.81,47.94 297.81,45.09 SV1.24
GPB1.0  (via drill 0.4)
  Top 0.254: v271.14,73.66 IC6.1
  Bottom 0.254: v271.14,73.66 271.14,72.39 276.54,66.99 276.54,65.72 281.31,60.96 SV1.9
GPB1.1  (via drill 0.4)
  Top 0.254: IC6.2 271.46,72.39 v272.73,73.66
  Bottom 0.254: v272.73,73.66 277.18,73.66 279.08,75.56 294.32,75.56 299.4,70.48 299.4,64.45 SV1.10
GPB1.2  (via drill 0.4)
  Top 0.254: v271.14,71.12 IC6.3
  Bottom 0.254: v271.14,71.12 271.14,70.48 283.21,58.42 SV1.11
GPB1.3  (via drill 0.4)
  Top 0.254: v267.97,69.85 IC6.4
  Bottom 0.254: v267.97,69.85 267.97,72.07 272.1,76.2 294.32,76.2 300.04,70.48 300.04,62.55 SV1.12
GPB1.4  (via drill 0.4)
  Top 0.254: v271.14,68.58 IC6.5
  Bottom 0.254: v271.14,68.58 272.42,68.58 285.12,55.88 SV1.13
GPB1.5  (via drill 0.4)
  Top 0.254: v271.14,67.31 IC6.6
  Bottom 0.254: v271.14,67.31 273.05,67.31 285.75,54.61 294.64,54.61 SV1.14
GPB1.6
  Top 0.254: IC6.7 274.95,66.04 278.13,62.87 280.35,62.87 289.56,53.66 292.42,53.66 292.74,53.34 SV1.15
GPB1.7  (via drill 0.4)
  Top 0.254: v271.14,64.77 IC6.8
  Bottom 0.254: v271.14,64.77 274.95,64.77 287.65,52.07 294.64,52.07 SV1.16
GPB2.0  (via drill 0.4)
  Top 0.254: IC7.1 267.65,46.99 267.33,46.67 267.33,42.23 268.29,41.27 270.51,41.27 271.78,40.01 272.73,40.01 276.23,36.51 277.18,36.51 278.13,37.47 280.35,37.47 v283.21,40.32
  Bottom 0.254: v283.21,40.32 293.05,40.32 SV1.25
GPB2.1
  Top 0.254: IC7.2 274.64,45.72 278.45,49.53 285.43,49.53 293.05,41.91 293.69,41.91 294.32,41.27 294.96,41.27 295.59,40.64 SV1.26
GPB2.2  (via drill 0.4)
  Top 0.254: IC7.3 268.92,44.45 268.29,43.81 268.29,42.55 275.27,42.55 v277.18,40.64
  Bottom 0.254: v277.18,40.64 278.13,40.64 280.67,38.1 SV1.27
GPB2.3
  Top 0.254: IC7.4 272.73,43.18 278.45,48.9 283.53,48.9 293.05,39.37 293.69,39.37 294.32,38.73 294.96,38.73 295.59,38.1 SV1.28
GPB2.4  (via drill 0.4)
  Top 0.254: IC7.5 272.1,41.91 v276.54,37.47
  Bottom 0.254: v276.54,37.47 277.81,36.2 292.74,36.2 SV1.29
GPB2.6  (via drill 0.4)
  Top 0.254: IC7.7 272.73,39.37 v276.54,35.56
  Bottom 0.254: v276.54,35.56 289.88,35.56 292.42,33.02 SV1.31
GPB2.7  (via drill 0.4)
  Top 0.254: IC7.8 272.42,38.1 v276.54,33.97
  Bottom 0.254: v276.54,33.97 290.83,33.97 293.05,31.75 294.64,31.75 SV1.32
GPIO1  (via drill 0.4)
  Top 0.203: v253.05,35.88 255.91,38.73 256.54,38.73 U$3.12
  Bottom 0.203: IC1.1 253.05,28.26 v253.05,35.88
GPIO2
  Top 0.203: IC1.2 249.87,26.67 254.63,31.43 254.63,35.88 256.54,37.78 257.18,37.78 258.13,38.73 258.13,39.37 259.08,40.32 259.08,41.27 U$3.13
GPIO3
  Top 0.203: IC1.3 249.87,29.21 252.09,31.43 252.09,35.88 256.22,40.01 256.86,40.01 258.13,41.27 258.13,41.91 259.08,42.86 259.08,43.81 U$3.15
GPIO4  (via drill 0.4)
  Top 0.203: v250.82,37.78 254,40.96 254,41.91 255.91,43.81 256.54,43.81 U$3.16
  Bottom 0.203: IC1.4 250.51,33.34 250.51,37.47 v250.82,37.78
GPIO5
  Top 0.203: IC1.5 249.87,34.29 254.63,39.05 254.63,41.27 256.22,42.86 257.18,42.86 258.13,43.81 258.13,44.77 256.54,46.35 U$3.18
GPIO6
  Top 0.203: IC1.6 247.97,36.83 244.16,40.64 244.16,42.86 248.92,47.62 252.09,47.62 255.91,51.44 256.54,51.44 U$3.22
GPIO7
  Bottom 0.203: IC1.7 250.51,39.37 254.95,34.92 254.95,33.97 256.22,32.7 258.13,32.7 259.08,33.66 U$3.7
GPIO21  (via drill 0.4)
  Top 0.203: IC1.8 249.56,41.91 v251.14,43.5
  Bottom 0.203: v251.14,43.5 251.14,55.24 256.54,60.64 258.13,60.64 259.08,61.59 U$3.29
GPIO27
  Top 0.203: T3.3 250.82,71.12 252.73,69.22 256.54,69.22 U$3.36
  Bottom 0.203: T3.3 250.19,72.07 251.14,73.03 251.14,79.06 R3.1
INT  (via drill 0.4)
  Top 0.406: K1.4 41.91,59.37 v49.53,66.99 | v143.83,73.66 157.48,60.01 R7.1
  Bottom 0.406: v49.53,66.99 59.69,66.99 66.36,73.66 v143.83,73.66 | IC3.21 218.12,50.8 213.68,55.24 213.68,60.01 212.41,61.28 159.38,61.28 153.99,55.88 153.35,55.88 152.4,54.93 152.4,54.29 153.99,52.7 155.57,52.7 R7.1
L
  Top 3.81: K17.P K17.P@ K12.P K12.P@ K8.P K8.P@ K16.P K16.P@ 95.57,28.89 90.49,23.81 K15.6 88.58,23.18 81.6,23.18 K15.3 79.69,23.18 73.98,23.18 K14.6 72.07,23.18 65.09,23.18 K14.3 63.18,23.18 57.47,23.18 K13.6 55.56,23.18 48.58,23.18 K13.3 46.67,22.23 46.04,21.59 37.15,21.59 27.94,30.8 27.94,31.43 26.99,33.02 | 26.99,33.02 D6.A 16.83,32.07 7.94,23.18 X1.1 | 26.99,33.02 27.94,33.97 C7.2
  Bottom 0.406: DCDC3.AC/L 164.22,51.2 158.75,45.72 158.75,43.18 K17.P
L-MOTOR
  Top 1.905: K13.4 48.58,18.1 55.56,18.1 K13.5
  Bottom 1.905: F1.2 48.26,17.78 K13.4
MISO  (via drill 0.4)
  Top 0.254: v269.24,29.53 269.24,30.48 IC7.14 | IC6.14 265.43,57.15 260.03,51.75 259.4,51.75 U$3.21
  Bottom 0.254: v269.24,29.53 269.24,30.48 267.02,32.7 267.02,35.88 260.35,42.55 260.35,50.48 259.4,51.44 U$3.21
MOSI
  Top 0.254: IC7.13 267.65,31.75 261.3,38.1 261.3,47.31 | 261.3,47.31 259.4,49.21 U$3.19 | IC6.13 269.88,58.42 270.83,57.47 270.83,56.83 261.3,47.31
N
  Bottom 0.406: DCDC3.AC/N 66.92,72 57.15,62.23 40.64,62.23 38.1,59.69 38.1,52.07 33.02,46.99 33.02,31.75 27.94,26.67 27.94,22.86 C7.1
  Bottom 3.81: 27.94,22.86 D6.C 16.83,21.91 13.02,18.1 7.94,18.1 X1.2
N$1
  Top 0.254: K1.2 28.57,55.24 28.57,66.99 30.16,68.58 T1.3
N$2
  Top 0.254: B1.- 7.62,46.99 11.43,50.8 D3.A 17.14,57.78 17.14,73.03 | T1.1 31.75,64.77 R9.1 | D1.A 17.78,72.39 17.14,73.03 | 17.14,73.03 C1.-
  Bottom 0.254: T1.1 30.16,66.04 25.4,70.8 D1.A
N$3
  Bottom 0.254: R1.1 14.92,59.69 12.38,62.23 11.43,62.23 | D2.C 11.43,62.23 | 11.43,62.23 C1.+
N$4
  Bottom 0.254: 22.86,48.26 19.05,44.45 R1.2 | 22.86,48.26 K1.1 | 22.86,48.26 D3.C
N$5
  Top 0.203: IC3.7 230.82,48.26 232.41,46.67 232.41,46.04 234.31,44.13 R13.2
N$6
  Top 0.203: LED1.A 234.95,37.15 233.36,37.15 233.04,37.47 233.04,40.32 R13.1
N$7
  Top 0.254: D1.C 25.4,60.96 R2.1
  Bottom 0.254: R4.2 22.86,73.66 22.86,67.31 D1.C
N$8  (via drill 0.4)
  Top 0.254: IC1.11 242.25,41.91 243.84,43.5 243.84,67.63 v241.3,70.17
  Bottom 0.254: v241.3,70.17 238.44,73.03 237.49,73.03 236.85,73.66 231.46,73.66 226.06,79.06 223.84,79.06 219.71,83.19 215.26,83.19 213.36,81.28 X6.3
N$9
  Top 0.254: T1.2 35.56,67.31 R9.2 R4.1
N$10
  Top 0.254: D2.A 4.76,51.75 4.76,39.69 7.62,36.83 B1.+
  Bottom 0.254: R2.2 21.91,41.91 16.83,36.83 7.62,36.83 B1.+
N$11
  Top 0.203: T3.2 245.43,75.25 245.43,77.79 245.11,78.11 R18.2
  Bottom 0.203: R18.2 240.66,83.19 228.6,83.19 226.69,81.28 223.52,81.28 X6.1
N$12  (via drill 0.6)
  Top 0.508: v87.63,63.5 T2.G
  Bottom 0.508: v87.63,63.5 82.87,58.74 63.82,58.74 K2.4
N$13
  Top 0.508: R5.1 71.12,55.88 K2.3
N$14  (via drill 0.4)
  Top 0.254: IC2.7 221.62,22.86 220.66,23.81 220.66,24.13 220.34,24.45 v220.34,25.4 | v216.85,32.38 216.85,31.43 218.44,29.84 R10.1
  Bottom 0.254: v220.34,25.4 220.34,27.3 R10.1 | IC3.13 231.78,61.59 231.78,45.4 230.5,44.13 228.6,44.13 223.52,39.05 219.39,39.05 218.12,37.78 217.81,37.78 216.85,36.83 v216.85,32.38
N$15  (via drill 0.4)
  Top 0.254: LED2.C 56.83,48.26 56.83,44.13 55.88,43.18 K13.8 | v246.7,43.81 v245.11,42.23 | v227.01,67.63 226.69,67.94 215.26,67.94 200.98,53.66 196.53,53.66 181.61,68.58 154.31,68.58 147.64,75.25 107,75.25 v101.28,65.72
  Bottom 0.254: IC1.18 244.16,26.99 244.16,41.27 v245.11,42.23 | v246.7,43.81 246.7,53.98 241.94,58.74 240.03,58.74 234.63,64.14 234.63,66.67 233.68,67.63 v227.01,67.63 | v101.28,65.72 93.34,65.72 71.44,45.09 57.78,45.09 55.88,43.18 K13.8
N$16  (via drill 0.4)
  Top 1.905: K7.3 170.5,23.18 177.48,23.18 K7.6 | B2.- 144.78,63.82 146.05,62.55 R15.1 146.69,54.29 157.48,43.5 157.48,42.55 v159.38,40.64
  Bottom 1.905: v159.38,40.64 165.1,34.92 165.1,28.26 170.18,23.18 K7.3
N$17
  Top 1.905: C2.1 48.26,62.23 R6.1
N$18  (via drill 0.9)
  Top 1.905: 48.26,70.17 44.45,73.98 L1.2 | C2.2 48.26,70.17 | v68.26,69.53 62.87,69.53 59.05,73.34 54.93,73.34 52.39,70.8 48.9,70.8 48.26,70.17
  Bottom 1.905: v68.26,69.53 124.14,69.53 129.54,64.14 B2.AC1
N$19  (via drill 0.4)
  Top 0.254: v225.11,32.38 224.47,31.75 v224.47,29.84
  Bottom 0.254: 229.87,22.54 IC2.1 C6.1 | IC3.2 228.28,35.56 v225.11,32.38 | v224.47,29.84 229.55,29.84 231.46,27.94 231.46,24.13 229.87,22.54 | 229.87,22.54 IC2.2
N$20
  Top 1.905: K9.5 193.99,18.1 187.01,18.1 K9.4 186.06,17.46 182.88,14.29 172.72,14.29 166.37,7.94 X4.2
N$21
  Top 1.905: K9.2 187.01,27.94 193.99,27.94 K9.7
  Bottom 1.905: D9.A 156.84,7.62 160.66,3.81 167.32,3.81 171.13,7.62 X4.3 172.09,7.94 181.61,17.46 181.61,22.86 186.69,27.94 K9.2
N$22
  Top 0.254: R11.1 LED2.A
N$23
  Top 1.422: T2.T1 82.55,78.74 81.92,79.38
  Top 1.905: D5.C 81.92,79.38 75.25,86.04 46.99,86.04 44.45,83.5 L1.1
N$24  (via drill 0.9)
  Top 1.905: D7.C 107.31,7.62 110.81,11.11 123.51,11.11 | 123.51,11.11 126.68,7.94 X5.1 | C4.1 143.19,44.45 128.27,59.37 124.14,59.37 119.7,63.82 B2.+ | 123.51,11.11 128.59,16.19 128.59,21.59 133.35,26.35 v139.06,26.35
  Bottom 1.905: v139.06,26.35 142.56,29.84 142.56,43.81 143.19,44.45 C4.1
N$25
  Top 0.203: IC3.9 230.5,53.34 233.68,50.16 C9.1
  Bottom 0.203: Q2.2 234.95,50.8 C9.1
N$26
  Top 0.203: IC3.10 230.82,55.88 234.95,60.01 Q2.1
  Bottom 0.203: C8.1 233.68,62.23 234.95,60.96 Q2.1
N$27  (via drill 0.4)
  Top 0.203: IC3.12 227.97,60.96 226.06,59.05 v225.11,59.05
  Bottom 0.203: v225.11,59.05 225.11,66.99 R12.1
N$28  (via drill 0.4)
  Top 0.254: v236.54,67.63 233.68,70.48 R17.1
  Bottom 0.254: C11.1 232.41,72.39 R17.1 | IC4.3 237.81,63.18 237.81,66.36 v236.54,67.63
N$29
  Top 0.254: IC4.4 240.35,57.15 238.44,59.05 238.44,70.17 238.76,70.48 R16.1
  Bottom 0.254: C12.1 241.94,69.22 240.66,69.22 R16.1 236.85,69.22 230.19,69.22 227.01,72.39 R12.2
N$30  (via drill 0.4)
  Top 0.254: K14.8 72.39,43.18 73.34,44.13 73.34,48.26 LED3.C 73.66,48.26 74.93,49.53 105.09,49.53 109.22,53.66 109.22,58.74 125.09,74.61 147.64,74.61 171.45,50.8 206.69,50.8 212.41,56.52 219.07,56.52 219.71,55.88 219.71,55.24 220.66,54.29 223.52,54.29 223.84,53.98 225.11,53.98 226.69,52.39 226.69,50.48 227.97,49.21 231.14,49.21 233.04,47.31 233.04,46.04 234,45.09 235.27,45.09 235.59,45.4 v237.81,43.18
  Bottom 0.254: IC1.17 239.08,28.89 239.08,41.91 v237.81,43.18
N$31
  Bottom 0.635: R14.1 119.38,45.72 R15.2
N$32
  Top 0.635: R14.2 116.2,44.45 119.06,47.31 125.41,47.31 128.27,44.45 C4.2
N$33
  Top 1.905: K9.6 193.99,23.18 187.01,23.18 K9.3 186.06,23.5 182.56,23.5 178.44,27.62 K7.7 177.48,27.94 170.5,27.94 K7.2 169.54,27.94 161.93,27.94 K6.7 160.97,27.94 153.99,27.94 K6.2
N$34
  Top 1.905: K7.4 170.5,18.1 177.48,18.1 K7.5
  Bottom 1.905: D9.C 145.1,7.62 153.67,16.19 153.67,17.78 K6.4 154.62,18.1 160.97,18.1 K6.5 | X4.1 161.29,7.94 161.29,17.14 K6.5 | K7.4 170.18,18.1 161.93,18.1 K6.5
N$35
  Top 1.905: K6.3 153.99,23.18 160.97,23.18 K6.6
  Bottom 1.905: D7.A 122.56,7.62 126.36,3.81 127.95,3.81 131.76,7.62 X5.2 132.72,8.26 135.57,11.11 144.15,11.11 149.54,16.51 149.54,18.73 153.67,22.86 K6.3
N$36
  Top 0.254: IC5.18 201.61,46.04 164.15,46.04 161.29,43.18 K6.8
N$37
  Bottom 0.254: R16.2 238.76,80.96 X3.1
N$38
  Bottom 0.254: R17.2 233.68,80.96 X3.2
N$39
  Top 0.254: C15.1 211.46,32.38 211.46,27.94 213.36,26.04 R20.2
  Bottom 0.254: IC2.6 220.03,23.18 220.03,20.95 218.76,19.68 215.26,19.68 R21.1 R20.2
N$40
  Top 0.254: R24.1 LED3.A
N$41
  Top 0.254: C13.1 217.81,34.29 216.85,33.34 216.53,33.34 215.9,32.7 215.9,28.57 218.44,26.04 R10.2
  Bottom 0.254: R23.2 228.28,15.24 | 228.28,15.24 R22.1 | R10.2 218.44,24.45 | 218.44,24.45 D10.C | 222.25,26.99 IC2.5 | 222.25,26.99 221.3,26.04 221.3,25.08 220.66,24.45 218.44,24.45 | 228.28,15.24 228.28,22.86 229.87,24.45 230.5,24.45 230.82,24.77 230.82,26.04 229.87,26.99 222.25,26.99
N$42  (via drill 0.4)
  Top 0.254: v102.87,34.61 103.82,35.56 LED4.C | IC1.16 242.25,29.21 246.38,25.08 246.38,23.18 v253.37,16.19 | v246.06,8.89 v247.65,10.48 | v169.54,2.54 160.97,2.54 147.64,15.88 145.41,15.88 138.75,22.54 v135.89,22.54
  Bottom 0.254: v102.87,34.61 101.28,33.02 101.28,23.18 K16.2 106.05,22.23 135.25,22.23 135.57,22.54 v135.89,22.54 | v247.65,10.48 v253.37,16.19 | v246.06,8.89 240.66,8.89 239.71,9.84 229.55,9.84 225.43,5.71 223.52,5.71 220.03,9.21 219.39,9.21 212.72,2.54 v169.54,2.54
N$43
  Bottom 0.254: U$3.31 259.08,64.45 258.13,64.45 256.86,65.72 256.22,65.72 251.78,70.17 251.78,80.01 244.16,87.63 214.63,87.63 208.28,81.28 X6.4
N$44  (via drill 0.4)
  Top 0.254: v247.01,82.87 247.01,77.79 247.97,76.83 250.19,76.83 256.22,70.8 256.86,70.8 258.13,69.53 259.08,69.53 U$3.35
  Bottom 0.254: v247.01,82.87 246.38,82.87 242.25,87 215.9,87 207.96,79.06 205.1,79.06 203.2,80.96 X6.5
N$45
  Top 0.254: R25.1 LED4.A
N$46
  Top 0.254: R26.1 LED5.A
N$49  (via drill 0.4)
  Top 0.254: 149.22,32.38 146.05,35.56 LED6.C | 149.22,32.38 149.22,23.5 K17.2 | IC1.13 237.81,36.83 236.22,35.24 v235.59,35.24 | v220.03,38.1 218.76,39.37 v218.76,39.69 | v212.09,38.42 208.28,34.61 151.45,34.61 149.22,32.38
  Bottom 0.254: v235.59,35.24 234.95,35.24 231.14,39.05 225.43,39.05 223.52,37.15 220.98,37.15 v220.03,38.1 | v218.76,39.69 213.36,39.69 v212.09,38.42
N$50
  Top 0.254: R27.1 LED6.A
N$51  (via drill 0.4)
  Top 0.254: v134.3,35.56 LED7.C | K12.2 v134.94,23.18 | v234.95,34.29 IC1.14 | v217.81,35.56 217.49,35.24 209.87,42.86 206.06,42.86 201.61,47.31 197.8,47.31 197.49,47.62 v156.84,47.62
  Bottom 0.254: v134.94,23.18 134.94,31.11 134.3,31.75 v134.3,35.56 134.3,38.73 143.19,47.62 v156.84,47.62 | v234.95,34.29 234.31,34.29 231.46,37.15 226.06,37.15 225.43,37.78 224.79,37.78 223.52,36.51 219.71,36.51 218.76,35.56 v217.81,35.56
N$52
  Top 0.254: R28.1 LED7.A
N$53  (via drill 0.4)
  Top 0.254: v116.84,34.61 117.79,35.56 LED8.C 118.11,35.56 122.24,39.69 141.6,39.69 145.73,43.81 145.73,45.09 140.97,49.85 140.97,64.45 143.83,67.31 145.1,67.31 148.27,64.14 148.27,59.05 148.91,58.42 148.91,57.78 153.99,52.7 157.16,52.7 159.07,54.61 167,54.61 172.72,48.9 197.49,48.9 197.8,48.58 201.93,48.58 202.25,48.9 v208.28,48.9 | K8.2 v115.25,23.18 | IC1.15 238.76,31.75 237.49,33.02 v234.95,33.02 | v225.11,36.83 225.43,37.15 225.43,40.96 v224.79,41.59
  Bottom 0.254: v116.84,34.61 115.25,33.02 v115.25,23.18 | v234.95,33.02 231.46,36.51 225.43,36.51 v225.11,36.83 | v224.79,41.59 217.49,41.59 214.31,44.77 211.77,44.77 208.28,48.26 v208.28,48.9
N$54
  Top 0.254: R29.1 LED8.A
N$55  (via drill 0.4)
  Top 0.254: LED5.C 89.85,48.26 89.85,44.13 88.9,43.18 K15.8 | v227.97,42.23 227.01,43.18 v227.01,43.81 | v209.55,48.26 209.23,47.94 197.8,47.94 197.49,48.26 159.38,48.26 v158.75,48.9
  Bottom 0.254: IC1.12 243.21,41.27 243.21,44.77 242.57,45.4 234.95,45.4 231.78,42.23 v227.97,42.23 | v227.01,43.81 225.11,43.81 223.52,42.23 219.07,42.23 215.9,45.4 212.09,45.4 209.55,47.94 v209.55,48.26 | v158.75,48.9 126.68,48.9 120.33,42.55 89.22,42.55 88.9,42.86 K15.8
N$57  (via drill 0.4)
  Top 0.203: v212.72,46.99 v209.87,44.13 | v224.47,46.99 225.43,47.94 225.43,48.58 v225.11,48.9 | v230.82,54.61 231.46,55.24 233.68,53.02 236.85,53.02 v238.76,51.12
  Bottom 0.203: IC5.2 202.25,38.1 205.74,34.61 208.28,34.61 209.87,36.2 v209.87,44.13 | v212.72,46.99 215.58,46.99 217.81,44.77 223.52,44.77 224.47,45.72 v224.47,46.99 | v225.11,48.9 225.11,50.8 228.6,54.29 230.5,54.29 v230.82,54.61 | v238.76,51.12 240.03,51.12 240.98,52.07 IC4.6
N$58
  Bottom 0.254: U$3.37 259.08,71.75 259.08,70.8 258.13,69.85 258.13,66.36 259.08,65.41 259.71,65.41 260.35,64.77 260.35,63.82 259.71,63.18 256.22,63.18 249.24,70.17 249.24,75.25 250.51,76.52 250.51,78.74 248.92,80.33 248.28,80.33 242.25,86.36 215.9,86.36 207.96,78.42 200.66,78.42 198.12,80.96 X6.6
N$60
  Top 0.254: IC5.17 201.61,38.1 200.03,39.69 198.12,39.69 196.22,41.59 196.22,44.45 195.26,45.4 180.02,45.4 177.8,43.18 K7.8
N$62
  Bottom 0.254: IC5.16 199.71,42.86 194.31,42.86 K9.8
N$63
  Top 3.81: K14.5 72.07,18.1 65.09,18.1 K14.4 64.45,16.19 52.39,4.13 24.45,4.13 21.59,6.99 21.59,7.62 20.32,8.89 X2.1
N$64  (via drill 0.4)
  Top 0.508: K16.S 93.66,14.92 73.34,14.92 v70.48,12.06
  Bottom 0.508: v70.48,12.06 28.26,12.06 25.4,9.21 X2.2
N$65  (via drill 0.4)
  Top 0.508: v47.94,13.97 35.24,13.97 30.48,9.21 X2.3
  Bottom 0.508: K8.S 107.63,14.92 103.19,14.92 99.38,18.73 99.38,21.27 89.53,31.11 55.56,31.11 51.44,26.99 51.44,17.46 v47.94,13.97
N$66  (via drill 0.4)
  Top 0.508: K12.S 120.02,13.34 76.52,13.34 72.39,9.21 v62.23,9.21
  Bottom 0.508: v62.23,9.21 45.72,9.21 X2.6
N$67  (via drill 0.4)
  Top 0.508: v53.66,14.92 50.8,12.06 43.5,12.06 40.64,9.21 X2.5
  Bottom 0.508: K17.S 131.76,11.11 91.44,11.11 82.23,20.32 78.11,20.32 72.71,14.92 v53.66,14.92
N$68
  Top 0.508: K15.4 81.6,18.1 88.58,18.1 K15.5
  Bottom 0.508: X2.4 35.56,8.89 38.73,5.71 69.22,5.71 81.28,17.78 K15.4
N$78  (via drill 0.6)
  other vias: 227.33,21.59
N_MOTOR
  Bottom 1.905: B1.AC2 7.62,41.59 3.49,37.47 3.49,16.19 6.67,13.02 7.62,13.02 X1.3 8.57,13.02 25.4,13.02 28.89,16.51 29.21,16.51 34.61,21.91 34.61,27.94 37.47,30.8 46.99,30.8 55.56,39.37 81.92,39.37 85.09,42.55 85.09,43.5 90.17,48.58 110.81,48.58 D5.A 124.14,54.61 128.91,59.37 132.72,59.37 137.16,63.82 B2.AC2
NTC
  Bottom 0.254: 201.93,13.97 C10.1 | R8.1 201.93,13.97 | IC2.3 225.43,20.95 225.43,8.89 226.06,8.26 226.06,6.99 225.43,6.35 223.52,6.35 220.03,9.84 213.68,9.84 209.55,5.71 201.29,5.71 199.39,7.62 X8.1 199.39,7.94 201.93,10.48 201.93,13.97
PGC  (via drill 0.4)
  Top 0.203: IC3.27 221.62,35.56 219.07,38.1 219.07,38.42 217.81,39.69 v217.81,45.72 | v210.19,55.56 208.6,57.15 208.6,60.33 211.77,63.5 v212.09,63.5
  Bottom 0.203: v217.81,45.72 217.81,46.35 214,50.16 214,51.75 v210.19,55.56 | v212.09,63.5 206.69,63.5 184.47,85.72 183.51,85.72 JP1.5
PGD  (via drill 0.4)
  Top 0.203: IC3.28 223.2,33.02 224.79,34.61 224.79,36.2 224.16,36.83 224.79,37.47 224.79,40.64 223.84,41.59 225.43,43.18 225.43,45.09 223.2,47.31 220.66,47.31 219.07,48.9 212.72,48.9 212.41,48.58 210.19,48.58 208.91,49.85 v205.74,49.85 | v191.45,60.33 177.16,74.61 177.16,80.33 179.07,82.23 JP1.4
  Bottom 0.203: v205.74,49.85 201.93,49.85 v191.45,60.33
PGM  (via drill 0.4)
  Top 0.203: IC3.26 221.3,38.1 219.71,39.69 v219.71,45.72 | v208.28,55.56 204.47,52.7 196.22,52.7 v184.15,64.77
  Bottom 0.203: v219.71,45.72 219.71,47.31 213.68,53.34 213.36,53.34 210.19,56.52 209.23,56.52 v208.28,55.56 | JP1.6 v184.15,64.77
PWM1
  Bottom 0.254: SV1.34 300.67,35.24 300.67,70.48 293.69,77.79 287.02,81.92 274.64,81.92 259.4,66.67 U$3.33
RX  (via drill 0.4)
  Top 0.254: IC3.18 223.2,58.42 v227.01,62.23
  Bottom 0.254: v227.01,62.23 227.01,62.87 228.6,64.45 231.14,64.45 232.41,63.18 232.41,49.21 235.59,46.04 242.57,46.04 248.28,40.32 250.19,40.32 256.54,33.97 U$3.8
SCK  (via drill 0.4)
  Top 0.254: v267.97,33.02 IC7.12 | v267.97,59.69 IC6.12
  Bottom 0.254: v267.97,33.02 267.97,35.56 260.99,42.55 260.99,52.7 | 260.99,52.7 259.4,54.29 U$3.23 | 260.99,52.7 v267.97,59.69
SCL  (via drill 0.4)
  Top 0.254: v247.01,11.43 245.43,9.84 237.17,9.84 234.95,7.62 X8.8
  Bottom 0.254: v247.01,11.43 247.97,11.43 252.41,15.88 252.41,26.04 256.22,29.84 256.86,29.84 258.13,31.11 259.08,31.11 U$3.5
SDA  (via drill 0.4)
  Top 0.254: v254.63,2.54 v259.08,6.99
  Bottom 0.254: v259.08,6.99 259.08,11.11 265.11,17.14 265.11,23.5 260.03,28.57 259.4,28.57 U$3.3 | v254.63,2.54 234.95,2.54 229.87,7.62 X8.7
SUPPLY_MOTOR
  Top 1.422: R5.2 87.63,58.42 85.09,60.96 T2.T2
  Top 1.905: B1.AC1 10.79,31.75 17.46,38.42 35.88,38.42 F1.1 | R5.2 76.52,55.88 73.03,52.39 66.67,52.39 64.45,54.61 R6.2
  Bottom 1.905: R6.2 52.07,54.61 F1.1
TACHO
  Bottom 0.254: 210.82,12.06 210.82,9.21 209.55,7.94 X8.3 | 210.82,12.06 C14.1 | R22.2 221.93,15.24 218.76,12.06 210.82,12.06
TRIAC  (via drill 0.4)
  Top 0.406: v214.63,55.56 v213.36,54.29
  Bottom 0.406: IC3.6 227.01,45.72 223.2,49.53 218.44,49.53 213.68,54.29 v213.36,54.29 | v214.63,55.56 214.63,60.01 212.72,61.91 183.51,61.91 169.23,76.2 K2.1
TX  (via drill 0.4)
  Top 0.254: IC3.17 223.2,60.96 v227.01,64.77
  Bottom 0.254: v227.01,64.77 227.97,64.77 228.28,65.09 231.14,65.09 233.04,63.18 233.04,61.28 238.76,55.56 242.57,55.56 245.75,52.39 245.75,43.5 246.38,42.86 250.19,42.86 256.54,36.51 U$3.10
VPP  (via drill 0.4)
  Top 0.203: IC3.1 231.78,33.02 234.95,36.2 236.54,36.2 238.76,38.42 238.76,50.16 239.71,51.12 237.81,53.02 237.81,68.58 v236.22,70.17 | v173.04,86.36 171.45,84.77 JP1.1
  Bottom 0.203: v236.22,70.17 233.36,73.03 229.55,73.03 228.6,73.98 227.65,73.98 219.07,82.55 216.53,82.55 211.77,77.79 200.66,77.79 199.39,79.06 192.41,79.06 185.1,86.36 v173.04,86.36

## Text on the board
tNames: +12 | OV | GND | S+ | S- | L | N | ROTOR | STATOR | NM | WashBerryPi 1.0 | OR | GR | BL | YE | PU | NTC | GND | T | T | 5V | 3V3 | SDA | SCL | GND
